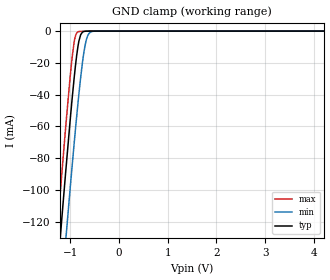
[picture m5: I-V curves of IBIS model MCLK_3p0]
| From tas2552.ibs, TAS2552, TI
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|   Model
[Model]   MCLK_3p0
Model_type   Input
Vinl = 0.9
Vinh = 2.1
|   typ   min   max
C_comp   1.014pF   0.983pF   1.069pF
[Voltage Range]   3   2.7   3.3
[Temperature Range]   27   125   -40
[Power Clamp Reference]   3   2.7   3.3
[GND Clamp Reference]   -0   -0   -0
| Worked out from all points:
|   GND clamp passes 1 mA (typ) near -0.76 V on its own axis
[GND Clamp]
|   Voltage   I(typ)   I(min)   I(max)
-3V       -843.1mA   -874.9mA   -823.7mA
-1.335V   -180.3mA   -222.6mA   -152.7mA
-1.173V   -118.6mA   -161.8mA   -90.27mA
-1.092V   -88.63mA   -131.9mA   -60.23mA
-957mV    -41.53mA   -83.83mA   -15.75mA
-894mV    -22.36mA   -62.51mA   -3.256mA
-840mV    -9.459mA   -45.24mA   -464.6uA
-786mV    -2.352mA   -29.44mA   -154uA
-696mV    -124.1uA   -9.252mA   -73.5uA
-633mV    -25uA      -2.445mA   -39.45uA
-552mV    -4.606uA   -280.5uA   -11.43uA
5.991V    0A         0A         0A
[POWER Clamp]
|   Voltage   I(typ)   I(min)   I(max)
-3V       0A         0A         0A
-2.982V   0A         0A         0A
-2.973V   0A         0A         0A
5.991V    0A         0A         0A
